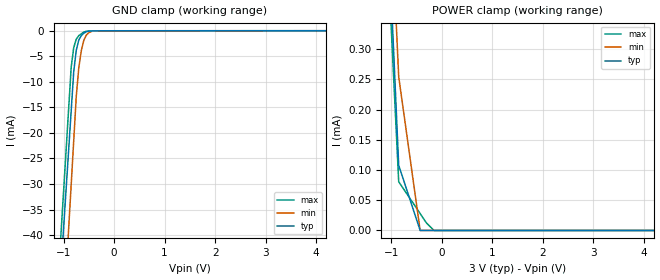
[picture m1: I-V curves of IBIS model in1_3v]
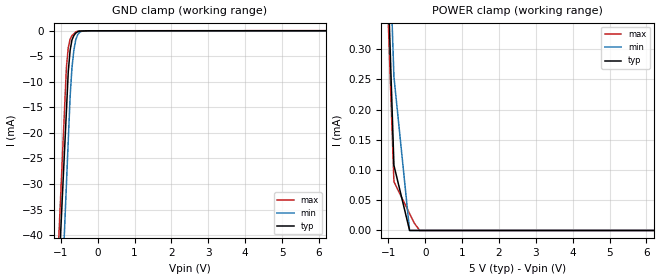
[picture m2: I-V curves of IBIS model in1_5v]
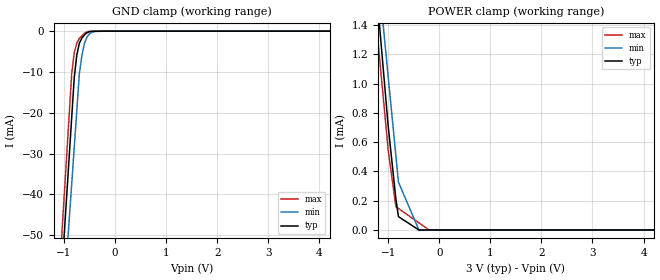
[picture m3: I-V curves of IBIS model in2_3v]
[IBIS Ver]   3.2
[Comment Char] |_char
[File Name]   dac8534ipw.ibs
[File Rev]   3.0
[Source]
| This model file was created by Teraspeed Consulting Group LLC
| (http://www.teraspeed.com/).
[Date]   09-13-2007
[Notes]   Quality Check of this IBIS model: Model Passes IBIS Check
   Model parses into ICX IS. Simulation done with Hyperlynx.
   1. MIN TYP MAX information is based on Temprature and Voltage
   characteristics only.
[Disclaimer]
| This model is designed as an aid for customers of Texas Instruments.
| TI and its licensors and suppliers make no warranties, either expressed
| or implied, with respect to this  model, including the warranties of
| merchantability or fitness for a particular purpose.
| The model is provided solely on an "as is" basis. The entire risk as to
| its quality and performance is with the customer.
[Copyright]
| (C) Copyright 2008 Texas Instruments Incorporated. All rights reserved.
[Component] DAC8534IPW
[Manufacturer] TI
[Package]
| variable   typ   min   max
R_pkg  1.602E-02   1.487E-02   1.721E-02
L_pkg  1.442E-09   1.338E-09   1.548E-09
C_pkg  4.006E-13   3.717E-13   4.301E-13
[Pin] signal_name  model_name  R_pin  L_pin C_pin
1   VOUT_A term   1.721E-02   1.548E-09   4.301E-13
2   VOUT_B term   1.640E-02   1.476E-09   4.100E-13
3   VREF_H term   1.562E-02   1.406E-09   3.905E-13
4   AVDD   POWER  1.487E-02   1.338E-09   3.717E-13
5   VREF_L term   1.487E-02   1.338E-09   3.717E-13
6   GND   GND   1.562E-02   1.406E-09   3.905E-13
7   VOUT_C term   1.640E-02   1.476E-09   4.100E-13
8   VOUT_D term   1.721E-02   1.548E-09   4.301E-13
9   _SYNC  in_1   1.721E-02   1.548E-09   4.301E-13
10   SCLK   in_1   1.640E-02   1.476E-09   4.100E-13
11   DIN   in_1   1.562E-02   1.406E-09   3.905E-13
12   IOVDD  POWER  1.487E-02   1.338E-09   3.717E-13
13   A0   in_1   1.487E-02   1.338E-09   3.717E-13
14   A1   in_1   1.562E-02   1.406E-09   3.905E-13
15   _EN   in_2   1.640E-02   1.476E-09   4.100E-13
16   LDAC   in_2   1.721E-02   1.548E-09   4.301E-13
[Model selector] in_1
in1_3v  3v input 1
in1_5v  5v input 1
[Model selector] in_2
in2_3v  3v input 2
in2_5v  5v input 2
[Model] term
Model_type Terminator
C_comp  0pF 0pF 0pF
| variable typ   min   max
[Voltage Range]   5.00000V  4.50000V  5.50000V
[POWER Clamp Reference]  5.00000V  4.50000V  5.50000V
[GND Clamp Reference]   0.00000V  0.00000V  0.00000V
[Temperature Range]   25   105   -40
| Models and submodels in the file (5): in1_3v (Input), in1_5v (Input), in2_3v (Input), in2_5v (Input), term (Terminator)
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[Model] in1_3v
Model_type Input
Vinl = 600.000mV
Vinh = 2.10000V
C_comp 2.00000pF 2.00000pF 2.00000pF
| variable typ   min   max
[Voltage Range] 3.00000V 2.70000V 3.30000V
[POWER Clamp Reference] 3.00000V 2.70000V 3.30000V
[GND Clamp Reference] 0.00000V 0.00000V 0.00000V
[Temperature Range]   25   105   -40
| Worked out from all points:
|   GND clamp passes 1 mA (typ) near -0.65 V on its own axis
[GND Clamp]
-5V       -649mA     -743mA     -676.5mA
-850mV    -15.64mA   -30.08mA   -7.105mA
-800mV    -8.009mA   -21.49mA   -3.29mA
-750mV    -3.825mA   -12.9mA    -1.659mA
-700mV    -1.809mA   -7.262mA   -946.7uA
-650mV    -960.6uA   -3.911mA   -603uA
-600mV    -475.5uA   -1.863mA   -259.4uA
-550mV    -204.5uA   -846.8uA   -83.71uA
-500mV    -66.21uA   -362.9uA   -68.59uA
-450mV    -53.15uA   -131.7uA   -53.46uA
-200mV    -888.9nA   -970.4nA   -249.2nA
10V       6.263uA    11.19uA    37.26uA
[POWER Clamp]
-5V       7.924mA    7.775mA    7.811mA
-1.4V     1.144mA    1.251mA    1.029mA
-850mV    107.8uA    254.6uA    80.77uA
-700mV    69.78uA    164.7uA    62.13uA
-425mV    0A         0A         27.96uA
-300mV    0A         0A         12.43uA
-150mV    0A         0A         0A
10V       0A         0A         0A
[Model] in1_5v
Model_type Input
Vinl = 800.000mV
Vinh = 2.40000V
C_comp 2.00000pF 2.00000pF 2.00000pF
| variable typ   min   max
[Voltage Range] 5.00000V 4.50000V 5.50000V
[POWER Clamp Reference] 5.00000V 4.50000V 5.50000V
[GND Clamp Reference] 0.00000V 0.00000V 0.00000V
[Temperature Range]   25   105   -40
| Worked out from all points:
|   GND clamp passes 1 mA (typ) near -0.65 V on its own axis
[GND Clamp]
-5V       -649mA     -743mA     -676.5mA
-850mV    -15.64mA   -30.08mA   -7.105mA
-800mV    -8.009mA   -21.49mA   -3.29mA
-750mV    -3.825mA   -12.9mA    -1.659mA
-700mV    -1.809mA   -7.262mA   -946.7uA
-650mV    -960.6uA   -3.911mA   -603uA
-600mV    -475.5uA   -1.863mA   -259.4uA
-550mV    -204.5uA   -846.8uA   -83.71uA
-500mV    -66.21uA   -362.9uA   -68.59uA
-450mV    -53.15uA   -131.7uA   -53.46uA
-200mV    -888.9nA   -970.4nA   -249.2nA
10V       6.263uA    11.19uA    37.26uA
[POWER Clamp]
-5V       7.924mA    7.775mA    7.811mA
-1.4V     1.144mA    1.251mA    1.029mA
-850mV    107.8uA    254.6uA    80.77uA
-700mV    69.78uA    164.7uA    62.13uA
-425mV    0A         0A         27.96uA
-300mV    0A         0A         12.43uA
-150mV    0A         0A         0A
10V       0A         0A         0A
[Model] in2_3v
Model_type Input
Vinl = 600.000mV
Vinh = 2.10000V
C_comp 2.00000pF 2.00000pF 2.00000pF
| variable typ   min   max
[Voltage Range] 3.00000V 2.70000V 3.30000V
[POWER Clamp Reference] 3.00000V 2.70000V 3.30000V
[GND Clamp Reference] 0.00000V 0.00000V 0.00000V
[Temperature Range]   25   105   -40
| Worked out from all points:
|   GND clamp passes 1 mA (typ) near -0.61 V on its own axis
[GND Clamp]
-5V       -833.8mA   -786.1mA   -855.4mA
-850mV    -21.2mA    -37.48mA   -10.47mA
-800mV    -11.41mA   -28.46mA   -5.251mA
-750mV    -5.806mA   -19.44mA   -2.945mA
-700mV    -2.959mA   -10.42mA   -1.792mA
-650mV    -1.695mA   -5.998mA   -1.149mA
-600mV    -888.5uA   -2.974mA   -505.5uA
-550mV    -392uA     -1.411mA   -163.1uA
-500mV    -126.7uA   -629.5uA   -33.48uA
-450mV    -27.92uA   -237.9uA   -26.94uA
-200mV    -1.028uA   -1.23uA    -659.6nA
10V       9.897uA    20.27uA    21.95uA
[POWER Clamp]
-5V       16.91mA    15.39mA    15.4mA
-1.4V     2.326mA    2.479mA    2.028mA
-1V       706uA      1.045mA    543.1uA
-850mV    212.3uA    506.6uA    159.5uA
-800mV    91.19uA    327.2uA    147.2uA
-700mV    68.39uA    245.4uA    122.7uA
-400mV    0A         0A         49.06uA
-300mV    0A         0A         24.53uA
-200mV    0A         0A         0A
-100mV    0A         0A         0A
10V       0A         0A         0A
